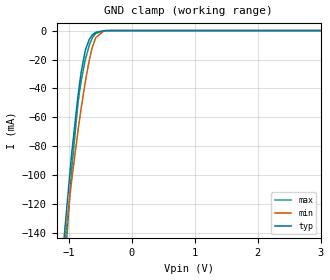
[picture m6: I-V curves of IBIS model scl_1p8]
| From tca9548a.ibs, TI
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|   scl_1p8 Model
[Model]   scl_1p8
Model_type   Input
Vinl = 0.54
Vinh = 1.26
|   typ   min   max
|   (nom PVT)   (fast PVT)   (slow PVT)
 C_comp   5.975e-12   5.695e-12   6.468e-12
[Model spec]
|subparameter
Vinl   0.54   0.513   0.567
Vinh   1.26   1.197   1.323
|Where nom  PVT is Nominal Process, 1.8V, 27C
|   Fast PVT is Strong Process,  1.89V, -40C
|   Slow PVT is Weak Process,   1.71V, 125C
[Voltage Range]   1.8   1.71   1.89
|Junction Temperature
[Temperature Range]   27   125   -40
[Power Clamp Reference]   1.8   1.71   1.89
[GND Clamp Reference]   0   0   0
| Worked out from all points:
|   GND clamp passes 1 mA (typ) near -0.55 V on its own axis
[GND Clamp]
|   Voltage   I(typ)   I(min)   I(max)
-1.8V     -583.7mA   -489.3mA   -734.8mA
-1.134V   -169.4mA   -171.2mA   -202.7mA
-966.5mV  -88.39mA   -106.3mA   -100.4mA
-860.7mV  -45.9mA    -69.99mA   -51.06mA
-808.2mV  -28.87mA   -53.71mA   -34.93mA
-739.7mV  -13.23mA   -34.65mA   -19.67mA
-676.5mV  -5.826mA   -19.93mA   -9.807mA
-630mV    -3.02mA    -11.5mA    -5.075mA
-573.9mV  -1.229mA   -4.78mA    -1.896mA
-450mV    -106.7uA   -333.5uA   -122.8uA
-367mV    -14.11uA   -48.47uA   -12.5uA
3.598V    0A         0A         0A
[POWER Clamp]
|   Voltage   I(typ)   I(min)   I(max)
-1.8V     0A         0A         0A
-1.49V    0A         0A         0A
3.598V    0A         0A         0A
